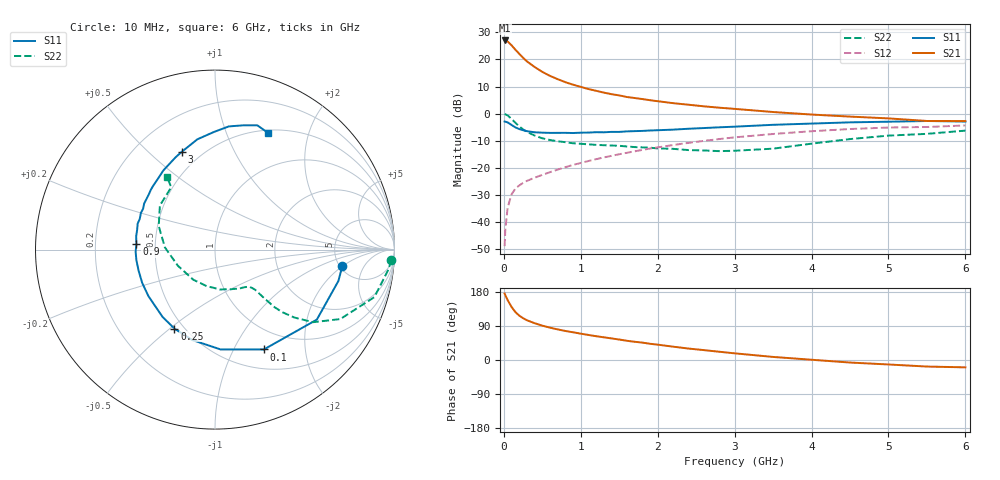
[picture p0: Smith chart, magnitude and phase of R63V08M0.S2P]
! SIEMENS Small Signal Semiconductors
! BFR193
! Si NPN RF Bipolar Junction Transistor in SOT23
! VCE = 3 V  IC = 8 mA
! Common Emitter S-Parameters:  May  1996
# GHz  S  MA  R  50
!  f  S11  S21  S12  S22
! GHz  MAG  ANG  MAG  ANG  MAG  ANG  MAG  ANG
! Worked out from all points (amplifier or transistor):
!   36 points, 10 MHz to 6 GHz, reference 50 ohm
!   highest |S21| = 27.0 dB at 10 MHz (marker M1)
!   |S21| within 3 dB of that: start of sweep to 137.5 MHz
!   unconditionally stable (mu >= 1): 796.9 MHz to 1.964 GHz
!   at 250 MHz: K = 0.57, MSG = 23.1 dB, |S12| = -25.5 dB
!   at 1.4 GHz: K = 1.05, MAG = 10.1 dB, |S12| = -15.6 dB
!   at 6 GHz: K = 0.95, MSG = 0.8 dB, |S12| = -4.4 dB
!   lowest NFmin = 1.25 dB at 450 MHz
!   S11 on the Smith chart (normalised r, x): 10 MHz: 5.29, -1.94; 100 MHz: 0.73, -1.33; 250 MHz: 0.45, -0.52; 900 MHz: 0.39, +0.03; 3 GHz: 0.39, +0.64; 6 GHz: 0.53, +1.42
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0.01  0.7154 -7.2  22.34 175.5  0.0036 86.0  0.985 -3.4
0.02  0.7095 -14.2  22.07 170.8  0.0075 86.2  0.9712 -6.8
0.05  0.6886 -34.5  21.34 157.8  0.0186 74.5  0.9265 -16.6
0.1  0.6194 -63.9  18.22 140.1  0.0324 63.6  0.7984 -29.0
0.15  0.5575 -86.7  15.09 126.5  0.0416 56.9  0.6799 -36.5
0.2  0.5194 -104.1  12.71 117.2  0.0473 54.5  0.5814 -40.6
0.25  0.4947 -117.2  10.69 110.3  0.0528 52.8  0.512 -42.9
0.3  0.475 -128.1  9.204 104.9  0.0575 53.2  0.4632 -44.0
0.4  0.4525 -145.1  7.243 97.1  0.0658 54.1  0.3941 -44.6
0.5  0.446 -155.5  5.883 90.7  0.0744 55.9  0.3506 -44.8
0.6  0.4415 -164.7  4.965 85.4  0.0833 57.2  0.3264 -44.8
0.7  0.4419 -172.3  4.316 80.7  0.0929 58.7  0.3096 -45.3
0.9  0.439 176.2  3.417 73.1  0.1135 60.4  0.2844 -47.0
1.1  0.4476 165.7  2.84 66.1  0.1338 61.1  0.2715 -50.1
1.3  0.4528 157.8  2.439 59.9  0.1559 60.9  0.2617 -54.2
1.6  0.4708 147.0  2.024 50.7  0.1899 59.8  0.248 -61.8
2.2  0.507 128.8  1.56 35.2  0.2637 55.0  0.2243 -82.8
3  0.5749 108.9  1.224 17.6  0.3651 44.7  0.2069 -125.7
3.5  0.6223 99.1  1.071 8.1  0.4216 37.1  0.226 -156.8
4.5  0.6906 83.6  0.882 -6.7  0.5202 21.6  0.3395 157.4
5.5  0.7314 71.2  0.732 -17.3  0.5673 5.7  0.424 125.1
6  0.7145 65.5  0.73 -19.4  0.6052 1.0  0.4861 123.4
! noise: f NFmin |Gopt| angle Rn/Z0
0.45  1.25  0.23  133  0.12
0.9  1.3  0.35  156  0.11
1.8  2  0.55  -155  0.13
